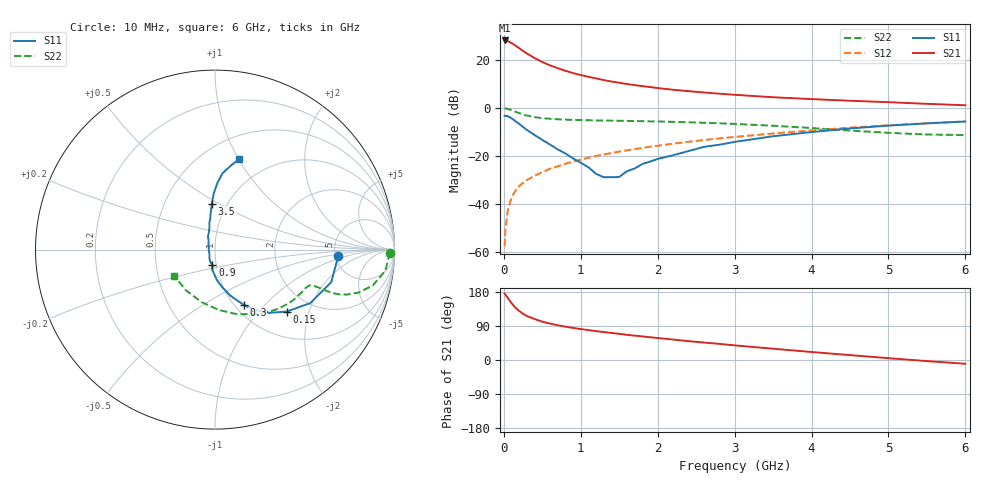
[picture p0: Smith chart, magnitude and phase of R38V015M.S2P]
! SIEMENS Small Signal Semiconductors
! BFR181
! Si NPN RF Bipolar Junction Transistor in SOT23
! VCE = 8 V  IC = 15 mA
! Common Emitter S-Parameters:  May  1996
# GHz  S  MA  R  50
!  f  S11  S21  S12  S22
! GHz  MAG  ANG  MAG  ANG  MAG  ANG  MAG  ANG
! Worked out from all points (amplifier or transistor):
!   36 points, 10 MHz to 6 GHz, reference 50 ohm
!   highest |S21| = 28.2 dB at 10 MHz (marker M1)
!   |S21| within 3 dB of that: start of sweep to 189.5 MHz
!   unconditionally stable (mu >= 1): 728.5 MHz to 2.639 GHz
!   at 250 MHz: K = 0.68, MSG = 27.5 dB, |S12| = -31.3 dB
!   at 1.4 GHz: K = 1.05, MAG = 13.5 dB, |S12| = -18.9 dB
!   at 6 GHz: K = 0.86, MSG = 3.4 dB, |S12| = -5.7 dB
!   S11 on the Smith chart (normalised r, x): 10 MHz: 5.31, -0.75; 150 MHz: 1.50, -1.44; 300 MHz: 1.10, -0.77; 900 MHz: 0.96, -0.17; 3.5 GHz: 0.85, +0.46; 6 GHz: 0.73, +1.00
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0.01  0.6885 -3.1  25.62 175.5  0.0013 85.4  0.9774 -1.1
0.02  0.6804 -6.3  25.44 172.5  0.0028 89.1  0.9679 -2.8
0.05  0.6727 -15.6  24.78 164.0  0.0071 80.8  0.956 -7.1
0.1  0.6089 -29.3  22.63 150.3  0.0135 77.8  0.9017 -12.8
0.15  0.5283 -40.8  20.11 137.8  0.0185 73.2  0.834 -16.7
0.2  0.4642 -49.4  17.65 129.2  0.0233 72.4  0.7772 -18.8
0.25  0.4006 -56.9  15.46 121.8  0.0273 70.1  0.7318 -19.9
0.3  0.346 -62.6  13.67 116.0  0.0313 70.7  0.694 -20.3
0.4  0.2725 -71.3  10.99 108.1  0.0384 70.8  0.6441 -20.3
0.5  0.2146 -79.0  9.062 101.1  0.0456 71.3  0.613 -20.1
0.6  0.1722 -86.0  7.749 96.1  0.0537 71.9  0.5933 -20.1
0.7  0.1363 -91.8  6.756 91.7  0.0604 72.2  0.5795 -20.2
0.9  0.0881 -99.3  5.343 84.7  0.076 72.0  0.5628 -20.8
1.1  0.0575 -123.0  4.466 79.0  0.0914 71.8  0.5526 -22.2
1.3  0.0357 -153.6  3.81 73.8  0.107 70.9  0.5452 -23.9
1.6  0.0477 139.0  3.151 66.4  0.1301 69.4  0.5356 -27.0
2.2  0.1028 109.3  2.396 53.9  0.1793 65.6  0.512 -34.8
3  0.1953 97.4  1.879 38.6  0.248 59.2  0.4642 -47.5
3.5  0.2564 94.0  1.671 29.8  0.2928 54.6  0.4244 -57.9
4.5  0.3727 87.9  1.413 12.9  0.3871 43.6  0.3366 -86.6
5.5  0.4758 79.4  1.218 -2.9  0.4782 31.1  0.2785 -125.4
6  0.5208 75.2  1.137 -10.0  0.5202 24.2  0.271 -147.5
